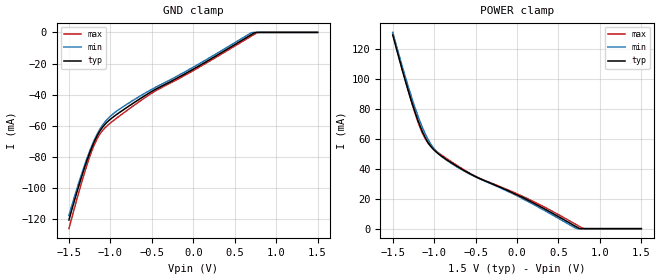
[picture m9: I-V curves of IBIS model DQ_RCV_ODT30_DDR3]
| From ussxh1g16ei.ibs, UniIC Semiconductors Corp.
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|   Model DQ_RCV_ODT30_DDR3
[Model] DQ_RCV_ODT30_DDR3
Model_type Input
Vinl =  0.615V
Vinh =  0.885V
C_comp   1.232pF   1.219pF   1.235pF
[Model Spec]
Vinh   0.885V   0.847V   0.922V
Vinl   0.615V   0.577V   0.652V
[Temperature Range]   25.000   95.000   -40.000
[Voltage Range]   1.500V   1.425V   1.575V
[GND_clamp]
|Voltage   I(typ)   I(min)   I(max)
-1.5V     -120.5mA   -117.7mA   -126.1mA
-1.345V   -92.36mA   -90.6mA    -96.06mA
-1.283V   -82.36mA   -80.98mA   -85.25mA
-1.221V   -73.53mA   -72.43mA   -75.74mA
-1.128V   -63.48mA   -62.29mA   -65.44mA
-1.066V   -59.1mA    -57.52mA   -61.36mA
-973mV    -54.65mA   -52.59mA   -57.07mA
-477mV    -37.21mA   -35.91mA   -38.27mA
-12mV     -23.99mA   -22.73mA   -24.92mA
701mV     -1.428mA   -226.9uA   -2.358mA
794mV     0A         0A         0A
1.5V      0A         0A         0A
[POWER_clamp]
|Voltage   I(typ)   I(min)   I(max)
-1.5V     129.5mA    131.1mA    131.2mA
-1.29V    88.13mA    90.97mA    87.89mA
-1.166V   68.05mA    70.99mA    66.95mA
-1.104V   60.49mA    62.96mA    59.7mA
-1.042V   55.11mA    56.69mA    55.11mA
-980mV    51.45mA    52.1mA     52.05mA
-887mV    47.49mA    47.32mA    48.29mA
-515mV    35.19mA    34.99mA    35.41mA
136mV     18.92mA    18.07mA    19.83mA
725mV     939uA      0A         2.381mA
818mV     0A         0A         0A
1.5V      0A         0A         0A
